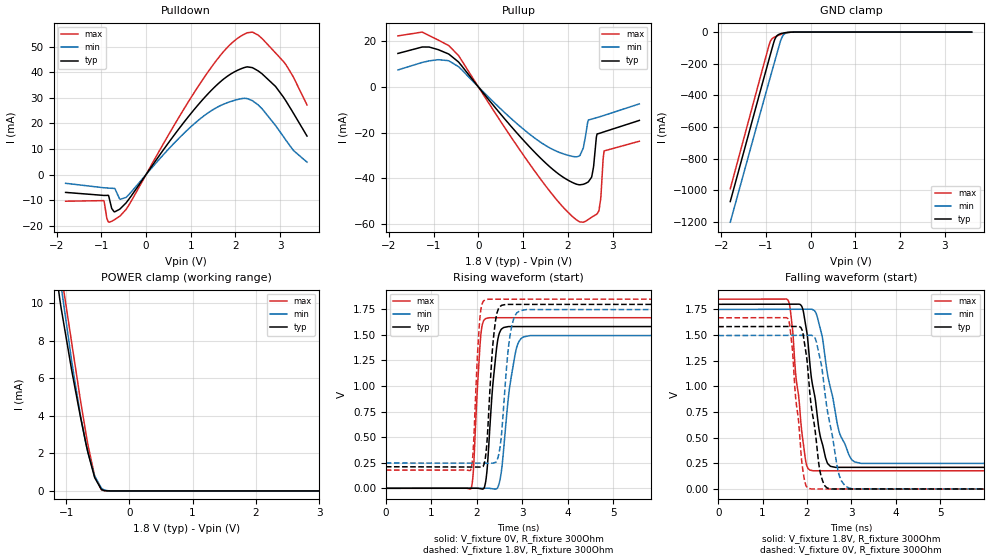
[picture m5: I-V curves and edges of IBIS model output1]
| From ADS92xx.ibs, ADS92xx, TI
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|   output1 Model
[Model]   output1
Model_type   3-state
Polarity   Non-Inverting
Vmeas = 0.9
Vref = 0
Cref = 2pF
Rref = 100000
|   typ   min   max
C_comp   0.480pF   0.471pF   0.482pF
[Voltage Range]   1.8   1.75   1.85
[Temperature Range]   27   125   -40
[Pullup Reference]   1.8   1.75   1.85
[Pulldown Reference]   0   0   0
[Power Clamp Reference]   1.8   1.75   1.85
[GND Clamp Reference]   0   0   0
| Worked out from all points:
|   slope of the pulldown table from 0 to 0.27 V, typ, clamps not added: 39.9 ohm
|   slope of the pullup table from 0 to 0.27 V, typ, clamps not added: 41.3 ohm
|   GND clamp passes 1 mA (typ) near -0.47 V on its own axis
|   POWER clamp passes 1 mA (typ) near -0.57 V on its own axis
|   falling waveform, V_fixture 1.8V, R_fixture 300Ohm: 20-80 % time 282ps typ, 375ps min, 214ps max; typ from 1.8 V to 0.21 V
|   rising waveform, V_fixture 0V, R_fixture 300Ohm: 20-80 % time 162ps typ, 225ps min, 117ps max; typ from 0 V to 1.58 V
|   rising waveform, V_fixture 1.8V, R_fixture 300Ohm: 20-80 % time 135ps typ, 169ps min, 107ps max; typ from 0.21 V to 1.8 V
|   falling waveform, V_fixture 0V, R_fixture 300Ohm: 20-80 % time 250ps typ, 321ps min, 192ps max; typ from 1.58 V to 0 V
[Pulldown]
|   Voltage   I(typ)   I(min)   I(max)
-1.8V     -6.967mA   -3.421mA   -10.41mA
-946.8mV  -8.149mA   -5.151mA   -10.18mA
-844.2mV  -8.109mA   -5.282mA   -18.45mA
-714.6mV  -14.53mA   -5.404mA   -17.71mA
-579.6mV  -13.39mA   -9.676mA   -16.14mA
-444.6mV  -11.02mA   -8.908mA   -13.58mA
1.37V     31.24mA    23.88mA    39.69mA
1.834V    38.58mA    28.17mA    49.95mA
2.266V    42.05mA    29.64mA    55.37mA
2.515V    40.39mA    27.07mA    54.33mA
3.071V    30.28mA    14.87mA    44.18mA
3.6V      15.03mA    4.843mA    27.19mA
[GND Clamp]
|   Voltage   I(typ)   I(min)   I(max)
-1.8V     -1.073A    -1.203A    -991.2mA
-1.071V   -314.5mA   -454mA     -226.1mA
-909mV    -148mA     -289.9mA   -62.37mA
-865.8mV  -104.1mA   -246.2mA   -41.84mA
-811.8mV  -51.82mA   -191.7mA   -31.75mA
-768.6mV  -27.09mA   -148.2mA   -26.27mA
-671.4mV  -10.22mA   -52.71mA   -15.1mA
-633.6mV  -7.364mA   -27.51mA   -11.3mA
-590.4mV  -4.79mA    -11.73mA   -7.529mA
-536.4mV  -2.452mA   -3.903mA   -3.915mA
-369mV    -68.54uA   -115.3uA   -98.1uA
3.6V      0A         0A         0A
[Pullup]
|   Voltage   I(typ)   I(min)   I(max)
-1.8V     14.68mA    7.438mA    22.38mA
-1.26V    17.48mA    10.72mA    24.04mA
-655.2mV  14.29mA    11.37mA    17.99mA
1.289V    -29.22mA   -22.84mA   -37.69mA
2.261V    -42.89mA   -30.2mA    -59.07mA
2.461V    -41.58mA   -14.49mA   -58.08mA
2.531V    -39.59mA   -14.13mA   -57.15mA
2.639V    -21.97mA   -13.5mA    -55.87mA
2.693V    -20.42mA   -13.2mA    -54.4mA
2.736V    -20.17mA   -12.95mA   -48.94mA
2.812V    -19.67mA   -12.47mA   -28.05mA
3.6V      -14.68mA   -7.428mA   -23.8mA
[POWER Clamp]
|   Voltage   I(typ)   I(min)   I(max)
-1.8V     31.2mA     30.7mA     34.65mA
-1.103V   10.28mA    11.52mA    12.11mA
-1.082V   9.796mA    10.98mA    11.66mA
-914.4mV  6.469mA    6.968mA    7.945mA
-774mV    3.948mA    4.022mA    4.832mA
-687.6mV  2.529mA    2.527mA    3.065mA
-655.2mV  2.04mA     2.046mA    2.454mA
-547.2mV  695.3uA    782.9uA    770.8uA
-439.2mV  77.91uA    141.2uA    59.78uA
-374.4mV  11.15uA    32.03uA    6.023uA
-261mV    173.7nA    1.498uA    26.38nA
3.6V      0A         0A         0A
[Ramp]
R_load = 300
|   typ   min   max
dV/dt_r   0.949593/1.61967e-10   0.897534/2.25287e-10   1.00122/1.16966e-10
dV/dt_f   0.953713/2.81424e-10   0.90161/3.74923e-10   1.00333/2.13544e-10
[Falling Waveform]
V_fixture = 1.8V
V_fixture_min = 1.75V
V_fixture_max = 1.85V
R_fixture = 300Ohm
C_fixture = 0F
|   Time   V(typ)   V(min)   V(max)
0s        1.8V       1.75V      1.85V
1.571ns   1.801V     1.752V     1.841V
1.908ns   1.748V     1.752V     470.4mV
1.99ns    1.542V     1.752V     233.2mV
2.135ns   988.2mV    1.746V     179.3mV
2.336ns   453mV      1.496V     179.3mV
2.467ns   247.2mV    1.105V     179.3mV
2.744ns   212.4mV    530.2mV    179.3mV
3.216ns   212.4mV    251mV      179.3mV
50ns      210.5mV    247.3mV    177.8mV
[Rising Waveform]
V_fixture = 0V
V_fixture_min = 0V
V_fixture_max = 0V
R_fixture = 300Ohm
C_fixture = 0F
|   Time   V(typ)   V(min)   V(max)
0s        1.14nV     11.7nV     5.808nV
1.873ns   456.1uV    481.4uV    -3.041mV
1.928ns   469.5uV    495.5uV    191.1mV
2.096ns   -5.512mV   538.7uV    1.527V
2.199ns   75.57mV    565.3uV    1.66V
2.271ns   477mV      32.79uV    1.667V
2.495ns   1.515V     52.5mV     1.667V
2.861ns   1.581V     1.348V     1.668V
3.176ns   1.581V     1.493V     1.668V
50ns      1.583V     1.496V     1.669V
[Rising Waveform]
V_fixture = 1.8V
V_fixture_min = 1.75V
V_fixture_max = 1.85V
R_fixture = 300Ohm
C_fixture = 0F
|   Time   V(typ)   V(min)   V(max)
0s        210.5mV    247.3mV    177.8mV
1.865ns   207.9mV    245.9mV    177.8mV
1.923ns   207.8mV    245.9mV    385.9mV
2.075ns   207.6mV    245.8mV    1.696V
2.25ns    643.3mV    245.6mV    1.849V
2.344ns   1.358V     245.6mV    1.849V
2.446ns   1.718V     276.6mV    1.849V
2.76ns    1.798V     1.564V     1.849V
3.102ns   1.798V     1.747V     1.849V
50ns      1.8V       1.75V      1.85V
[Falling Waveform]
|Gnd
V_fixture = 0V
V_fixture_min = 0V
V_fixture_max = 0V
R_fixture = 300Ohm
C_fixture = 0F
|   Time   V(typ)   V(min)   V(max)
0s        1.583V     1.496V     1.669V
1.571ns   1.584V     1.497V     1.659V
1.669ns   1.584V     1.498V     1.364V
1.891ns   1.547V     1.498V     232.9mV
2.096ns   805.6mV    1.498V     1.471mV
2.211ns   455.2mV    1.432V     1.467mV
2.375ns   54.29mV    1.039V     1.462mV
2.72ns    2.033mV    140.6mV    1.452mV
3.067ns   2.018mV    2.451mV    1.441mV
50ns      1.138nV    11.7nV     5.808nV
